|Texas Instruments Incorporated
|Octal, Low Power, 14-Bit, +/-16.5V Output Parallel Input Digital-To-Analog
|Converter
| Marketing part#   Digital Voltage Range   Package-type   #pins
| DAC8228SPAG   1.7V to 5.5V   TQFP   64
| DAC8228SPAGR   1.7V to 5.5V   TQFP   64
| DAC8228SRTQR   1.7V to 5.5V   QFN   56
| DAC8228SRTQT   1.7V to 5.5V   QFN   56
[IBIS Ver]   3.2
[File name]   dac8228.ibs
|SIMDE Ver   V2.2 - 201009 - RHL4 - Build 424
[File Rev]   1.1
[Date]   02/24/2011
[Source]
| Texas Instruments Incorporated.
| Analog-eLab Design Center, HPA
| 12500 TI Blvd
| Dallas, TX -75243
| e-mail: elab_ibis@list.ti.com
| -Model generated from simulations in TISPICE
[Notes]   Revision History:
| Rev 1.0: 02/02/2011
| - Initial version of the model
| - Model generated from simulations in TISPICE
| - Model matched to SPICE simulation
| - C_comp although listed in numerical order of value are
|   obtained from varying PVT conditions. For PVT conditions for
|   each specific value refer the buffer description under
|   respective [Model]. IBIS model user is responsible for using
|   appropriate C_comp to simulate for Signal Integrity.
| - Model names with a trailing _1p8 contains the model for
|   1.8V [1.71V and 1.89V].Model names with a trailing _3p3 contains
|   the model for 3.3V [3.0V and 3.6V]. Model names with trailing _5
|   contains the model for 5.0V [4.5V and 5.5V] operation.
| - Rleative of DAC8728
| Rev 1.1: 02/24/2011
| - Updated the Cref value for open_drain and io buffers.
| - Updated the R_fixture for open_drain buffers.
[Disclaimer]
| This model is designed as an aid for customers of Texas Instruments.
| TI and its licensors and suppliers make no warranties, either expressed
| or implied, with respect to this  model, including the warranties of
| merchantability or fitness for a particular purpose. The model is
| provided solely on an "as is" basis. The entire risk as to its quality
| and performance is with the customer.
[Copyright]
 (C) Copyright 2011 Texas Instruments Incorporated.All rights reserved.
|   DAC8228RTQ
[Component]   DAC8228RTQ
[Manufacturer]   TI
[Package]   |56 QFN  -  RTQ package
|   typ   min   max
R_pkg   0.09068   0.05574   0.13940
L_pkg   1.64354nH   1.39247nH   2.54711nH
C_pkg   0.21828pF   0.19939pF   0.32504pF
[Pin]  signal_name   model_name   R_pin   L_pin   C_pin
1   D13   DATA   0.09959   1.79067nH  0.20526pF
2   D14   DATA   0.09017   1.59422nH  0.21705pF
3   D15   DATA   0.08511   1.49967nH  0.20798pF
4   VMON   TERM   0.08460   1.49003nH  0.20659pF
5   VOUT-3   TERM   0.08300   1.46133nH  0.20788pF
6   REF-A   TERM   0.08502   1.49991nH  0.20848pF
7   VOUT-2   TERM   0.08516   1.50251nH  0.20857pF
8   AVDD   POWER   0.04488   1.15500nH  0.26176pF
9   AGND-A   GND   0.04584   1.21458nH  0.26686pF
10   VOUT-1   TERM   0.09839   1.74975nH  0.23512pF
11   AVSS   POWER   0.05458   1.53547nH  0.28939pF
12   OFFSET-A   TERM   0.05574   1.57953nH  0.28920pF
13   VOUT-0   TERM   0.11777   2.11608nH  0.24634pF
14   _USB/BTC   USB_RST   0.10115   1.82766nH  0.20568pF
15   _BUSY   BUSY   0.09644   1.73961nH  0.20115pF
16   _CLR   INPUT   0.08737   1.54876nH  0.20986pF
17   _LDAC   INPUT   0.08250   1.45720nH  0.20410pF
18   _RST   INPUT   0.08266   1.45974nH  0.20372pF
19   A0   INPUT   0.07986   1.40841nH  0.20209pF
20   A1   INPUT   0.07899   1.39247nH  0.20241pF
21   DVDD   POWER   0.04018   0.95363nH  0.25294pF
22   DGND   GND   0.04028   0.94247nH  0.25408pF
23   A2   INPUT   0.07903   1.39317nH  0.20104pF
24   A3   INPUT   0.07913   1.39514nH  0.19962pF
25   A4   INPUT   0.08000   1.41105nH  0.19939pF
26   DGND   GND   0.07911   1.39527nH  0.19893pF
27   GPIO   GPIO   0.08630   1.52941nH  0.21289pF
28   RSTSEL   USB_RST   0.10436   1.88898nH  0.21302pF
29   VOUT-7   TERM   0.13940   2.54711nH  0.25591pF
30   OFFSET-B   TERM   0.06564   1.95159nH  0.32504pF
31   AVSS   POWER   0.06428   1.89573nH  0.32497pF
32   VOUT-6   TERM   0.11576   2.07584nH  0.26261pF
33   AGND-B   GND   0.05306   1.46662nH  0.29405pF
34   AVDD   POWER   0.05137   1.37045nH  0.28459pF
35   VOUT-5   TERM   0.09565   1.69845nH  0.22183pF
36   REF-B   TERM   0.09540   1.69384nH  0.22071pF
37   VOUT-4   TERM   0.08740   1.54456nH  0.21024pF
38   NC   NC   0.00125   0.17541nH  0.12112pF
39   D0   DATA   0.08366   1.47467nH  0.20543pF
40   D1   DATA   0.08364   1.47321nH  0.20917pF
41   D2   DATA   0.08760   1.54720nH  0.21102pF
42   D3   DATA   0.10702   1.93238nH  0.21141pF
43   D4   DATA   0.11545   2.08793nH  0.22549pF
44   D5   DATA   0.10448   1.85950nH  0.23633pF
45   D6   DATA   0.09477   1.67625nH  0.22490pF
46   DGND   GND   0.04687   1.16167nH  0.27351pF
47   IOVDD   POWER   0.08786   1.54722nH  0.21661pF
48   DVDD   POWER   0.04353   1.02545nH  0.26376pF
49   R/_W   INPUT   0.08885   1.56550nH  0.21386pF
50   _CS   INPUT   0.08210   1.44056nH  0.20728pF
51   D7   DATA   0.07954   1.39337nH  0.20321pF
52   D8   DATA   0.08055   1.41215nH  0.20390pF
53   D9   DATA   0.08439   1.48309nH  0.20679pF
54   D10   DATA   0.08691   1.53035nH  0.21037pF
55   D11   DATA   0.09398   1.66365nH  0.22151pF
56   D12   DATA   0.10458   1.88554nH  0.21155pF
|   DAC8228PAG
[Component]   DAC8228PAG
[Manufacturer]   TI
[Package]   |64 TQFP  -  PAG package
|   typ   min   max
R_pkg   0.10033   0.05701   0.10904
L_pkg   3.36815nH   3.03842nH   3.68738nH
C_pkg   0.49998pF   0.43598pF   0.54508pF
[Pin]  signal_name   model_name   R_pin   L_pin   C_pin
1   D13   DATA   0.10566   3.62723nH  0.46020pF
2   D14   DATA   0.10159   3.45743nH  0.53671pF
3   D15   DATA   0.10000   3.35720nH  0.52701pF
4   VMON   TERM   0.10176   3.34678nH  0.50918pF
5   VOUT-3   TERM   0.10148   3.31393nH  0.50571pF
6   REF-A   TERM   0.10162   3.25664nH  0.48357pF
7   VOUT-2   TERM   0.10253   3.21700nH  0.47296pF
8   AVDD   POWER   0.05640   2.85004nH  0.48401pF
9   AGND-A   GND   0.05640   2.88385nH  0.48599pF
10   VOUT-1   TERM   0.10476   3.25937nH  0.48540pF
11   AVSS   POWER   0.05793   3.01181nH  0.53297pF
12   OFFSET-A   TERM   0.05701   3.03907nH  0.54508pF
13   VOUT-0   TERM   0.10486   3.40621nH  0.51117pF
14   NC   NC   0.00952   1.99807nH  0.43931pF
15   _USB/BTC   USB_RST   0.09971   3.42490nH  0.52978pF
16   _BUSY   BUSY   0.10261   3.57554nH  0.45689pF
17   _CLR   INPUT   0.10804   3.67674nH  0.46169pF
18   _LDAC   INPUT   0.10384   3.50383nH  0.53542pF
19   _RST   INPUT   0.10820   3.51169nH  0.53466pF
20   A0   INPUT   0.10606   3.43047nH  0.51577pF
21   A1   INPUT   0.10458   3.37513nH  0.50308pF
22   NC   NC   0.00916   1.86104nH  0.39171pF
23   NC   NC   0.00889   1.80020nH  0.38069pF
24   DVDD   POWER   0.05377   2.70150nH  0.47681pF
25   DGND   GND   0.05395   2.69082nH  0.48509pF
26   A2   INPUT   0.09806   3.14045nH  0.46810pF
27   A3   INPUT   0.09732   3.18322nH  0.47406pF
28   NC   NC   0.00943   1.92658nH  0.41197pF
29   A4   INPUT   0.09635   3.25388nH  0.49904pF
30   DGND   GND   0.09406   3.25402nH  0.51527pF
31   NC   NC   0.00979   2.07445nH  0.44475pF
32   NC   NC   0.00986   2.17258nH  0.36899pF
33   GPIO   GPIO   0.10262   3.57573nH  0.45600pF
34   RSTSEL   USB_RST   0.09972   3.42583nH  0.52906pF
35   NC   NC   0.00952   1.99850nH  0.43874pF
36   VOUT-7   TERM   0.10486   3.40638nH  0.51087pF
37   OFFSET-B   TERM   0.05701   3.03842nH  0.54504pF
38   AVSS   POWER   0.05792   3.01056nH  0.53313pF
39   VOUT-6   TERM   0.10476   3.25940nH  0.48545pF
40   AGND-B   GND   0.05640   2.88225nH  0.48609pF
41   AVDD   POWER   0.05640   2.85149nH  0.48388pF
42   VOUT-5   TERM   0.10253   3.21717nH  0.47285pF
43   REF-B   TERM   0.10163   3.25742nH  0.48288pF
44   VOUT-4   TERM   0.10149   3.31419nH  0.50108pF
45   NC   NC   0.00937   1.95351nH  0.41976pF
46   D0   DATA   0.10000   3.35687nH  0.52714pF
47   D1   DATA   0.10262   3.47520nH  0.53964pF
48   D2   DATA   0.10716   3.65444nH  0.46174pF
49   D3   DATA   0.10605   3.63275nH  0.45770pF
50   D4   DATA   0.10554   3.52693nH  0.53845pF
51   D5   DATA   0.10218   3.39359nH  0.53245pF
52   D6   DATA   0.09950   3.30245nH  0.50826pF
53   NC   NC   0.00943   1.92643nH  0.41193pF
54   DGND   GND   0.05428   2.78415nH  0.52691pF
55   IOVDD   POWER   0.09831   3.13580nH  0.47407pF
56   DVDD   POWER   0.05443   2.69518nH  0.48680pF
57   R/_W   INPUT   0.09969   3.15690nH  0.43598pF
58   _CS   INPUT   0.09829   3.13555nH  0.47210pF
59   D7   DATA   0.09855   3.19662nH  0.48223pF
60   D8   DATA   0.09979   3.27938nH  0.50309pF
61   D9   DATA   0.10124   3.33408nH  0.51014pF
62   D10   DATA   0.10041   3.36062nH  0.52890pF
63   D11   DATA   0.10336   3.48625nH  0.53916pF
64   D12   DATA   0.10904   3.68738nH  0.46353pF
|   Model Selectors
[Model Selector] INPUT
input_1p8  1.8V digital input
input_3p3  3.3V digital input
input_5   5.0V digital input
[Model Selector] USB_RST
usb_rst_1p8   1.8V digital input
usb_rst_3p3   3.3V digital input
usb_rst_5   5.0V digital input
[Model Selector] DATA
data_1p8   1.8V digital I/O
data_3p3   3.3V digital I/O
data_5   5.0V digital I/O
[Model Selector] GPIO
gpio_1p8   1.8V digital I/O_open_drain
gpio_3p3   3.3V digital I/O_open_drain
gpio_5   5.0V digital I/O_open_drain
[Model Selector] BUSY
busy_1p8   1.8V digital Open_drain
busy_3p3   3.3V digital Open_drain
busy_5   5.0V digital Open_drain
[Model Selector] TERM
term_1-8V  1.8V nominal termination
term_3-3V  3.3V nominal termination
term_5-0V  5.0V nominal termination
[Model]  term_1-8V
Model_type Terminator
C_comp   1.0e-20F  1.0e-20F  1.0e-20F
|   typ   min   max
[Voltage Range]   1.8V   1.71V   1.89V
[POWER Clamp Reference]   1.8V   1.71V   1.89V
[GND Clamp Reference]   0V   0V   0V
|Ambient Temperature   25   105   -40
|Junction Temperature
[Temperature Range]   33   113   -40
[Model]  term_3-3V
Model_type Terminator
C_comp   1.0e-20F  1.0e-20F  1.0e-20F
|   typ   min   max
[Voltage Range]   3.3V   3.0V   3.6V
[POWER Clamp Reference]   3.3V   3.0V   3.6V
[GND Clamp Reference]   0V   0V   0V
|Ambient Temperature   25   105   -40
|Junction Temperature
[Temperature Range]   33   113   -40
[Model]  term_5-0V
Model_type Terminator
C_comp   1.0e-20F  1.0e-20F  1.0e-20F
|   typ   min   max
[Voltage Range]   5.0V   4.5V   5.5V
[POWER Clamp Reference]   5.0V   4.5V   5.5V
[GND Clamp Reference]   0V   0V   0V
|Ambient Temperature   25   105   -40
|Junction Temperature
[Temperature Range]   33   113   -40
| Models and submodels in the file (18): input_1p8 (Input), input_3p3 (Input), input_5 (Input), usb_rst_1p8 (Input), usb_rst_3p3 (Input), usb_rst_5 (Input), data_1p8 (I/O), data_3p3 (I/O), data_5 (I/O), gpio_1p8 (I/O_open_drain), gpio_3p3 (I/O_open_drain), gpio_5 (I/O_open_drain), busy_1p8 (Open_drain), busy_3p3 (Open_drain), busy_5 (Open_drain), term_1-8V (Terminator), term_3-3V (Terminator), term_5-0V (Terminator)
